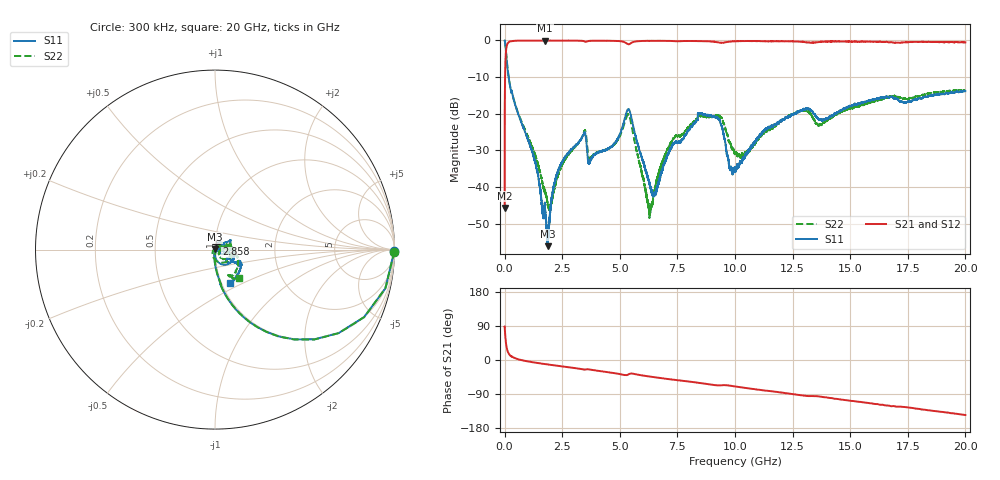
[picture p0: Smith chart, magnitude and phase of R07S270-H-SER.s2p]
!{R07S270}
!Johanson Technology Inc.
!www.johansontechnology.com
!Test Board Conditions:
!Substrate Type  RO4350B
!Substrate Thickness  10 mil
!Substrate Dk  3.66
!TL Type: GCPW
!TL Trace Width  21 mil
!TL Gap  20 mil
!Electrode orientation  Horizontal
!DUT TOPOLOGY	SERIES
!Mounting Pad LxW  16x21 mil
! Created Sat Feb  6 11:53:17 2021
# hz S ma R 50
! 2 Port Network Data from SP1.SP block
! freq  magS11  angS11  magS21  angS21  magS12  angS12  magS22  angS22
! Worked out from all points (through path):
!   20001 points, 300 kHz to 20 GHz, reference 50 ohm
!   highest |S21| = -0.02 dB at 1.754 GHz (marker M1); lowest = -45.7 dB at 300 kHz (marker M2)
!   group delay of S21, straight-line fit = 20.7 ps
!   lowest |S11| = -56.1 dB at 1.879 GHz (marker M3), VSWR 1.00, Z = 49.9 + j0.0689 ohm
!   |S11| at or under -10 dB: 176.1 MHz to end of sweep
!   |S22| runs from -48.5 to 0.0 dB; largest |S21 - S12| = 0.013
!   S11 on the Smith chart (normalised r, x): 300 kHz: open; 2.858 GHz: 1.01, +0.06; 20 GHz: 1.09, -0.42
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300000  0.9982 -0.6  0.005175 88.6  0.005258 88.4  0.9993 -0.7
1.023e8  0.4971 -61.0  0.8642 29.3  0.8659 29.2  0.4986 -60.9
1.573e8  0.3501 -71.0  0.9348 19.4  0.935 19.4  0.3491 -70.8
1.3143e9  0.02253 -102.3  0.9967 -6.8  0.9965 -6.8  0.0282 -89.9
1.7543e9  0.004888 -118.3  0.9979 -10.7  0.997 -10.7  0.00906 -74.4
1.8793e9  0.001558 153.7  0.997 -11.8  0.9962 -11.8  0.005586 -43.3
2.2273e9  0.01358 84.9  0.9968 -14.7  0.9961 -14.7  0.01183 40.4
2.8583e9  0.03175 75.2  0.9945 -19.8  0.9936 -19.8  0.0302 52.0
3.3343e9  0.0457 62.9  0.9885 -23.9  0.9893 -23.9  0.04615 49.3
3.7153e9  0.02252 49.7  0.9864 -25.4  0.9871 -25.4  0.02494 34.2
4.7673e9  0.03891 36.4  0.9862 -34.6  0.9853 -34.7  0.03819 55.4
5.3833e9  0.1151 -33.8  0.887 -37.8  0.887 -37.8  0.09726 -33.9
6.2603e9  0.0121 -69.7  0.9871 -43.3  0.988 -43.3  0.005074 157.4
6.6673e9  0.01086 17.9  0.9874 -46.7  0.9883 -46.8  0.01424 48.9
7.3473e9  0.03968 33.5  0.9795 -52.3  0.9793 -52.3  0.04618 21.2
8.4873e9  0.09968 31.0  0.9781 -60.8  0.9784 -60.8  0.09309 22.9
9.2903e9  0.08451 -1.0  0.9383 -67.0  0.9392 -67.1  0.09595 -18.3
1.00003e10  0.01731 4.8  0.9747 -69.8  0.9759 -69.8  0.02835 -44.5
1.13773e10  0.06279 -17.5  0.9741 -81.1  0.9738 -81.1  0.05835 6.7
1.33343e10  0.1087 -42.1  0.9308 -95.1  0.932 -95.2  0.09379 -21.8
1.66673e10  0.166 -29.9  0.9406 -120.3  0.9449 -120.7  0.1699 -46.5
2e10  0.2035 -66.5  0.9425 -145.3  0.937 -145.2  0.2058 -50.2
